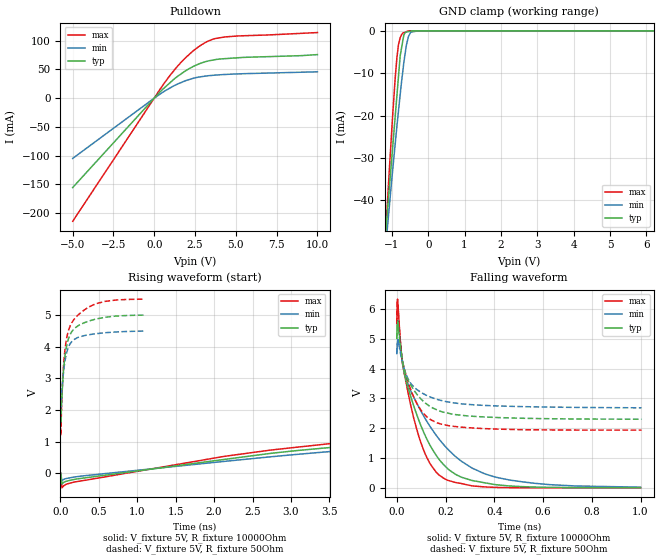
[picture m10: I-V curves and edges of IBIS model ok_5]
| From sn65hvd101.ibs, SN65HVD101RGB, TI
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|   ok_5 Model
[Model]   ok_5
Model_type   Open_drain
Polarity   Inverting
Vmeas = 2.5
Vref = 5
Cref = 2pF
Rref = 10000
|   typ   min   max
|   (nom PVT)   (fast PVT)   (slow PVT)
C_comp   1.593e-12   1.577e-12   1.617e-12
| Where nom  PVT is Nominal Process, 5V, 45C
|   Fast PVT is Strong Process,  5.5V, -20C
|   Slow PVT is Weak Process,   4.5V, 125C
[Voltage Range]   5   4.5   5.5
|Junction Temperature
[Temperature Range]   45   125   -20
[Pullup Reference]   5   4.5   5.5
[Pulldown Reference]   0   0   0
[Power Clamp Reference]   5   4.5   5.5
[GND Clamp Reference]   0   0   0
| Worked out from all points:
|   slope of the pulldown table from 0 to 0.75 V, typ, clamps not added: 35.3 ohm
|   GND clamp passes 1 mA (typ) near -0.67 V on its own axis
|   falling waveform, V_fixture 5V, R_fixture 10000Ohm: 20-80 % time 142ps typ, 220ps min, 98.9ps max; typ from 5 V to 0.017 V
|   rising waveform, V_fixture 5V, R_fixture 10000Ohm: 20-80 % time 27.8ns typ, 28.8ns min, 27.6ns max; typ from 0.016 V to 5 V
|   falling waveform, V_fixture 5V, R_fixture 50Ohm: 20-80 % time 97.8ps typ, 111ps min, 79.6ps max; typ from 5 V to 2.31 V
|   rising waveform, V_fixture 5V, R_fixture 50Ohm: 20-80 % time 115ps typ, 104ps min, 133ps max; typ from 2.31 V to 4.99 V
[Pulldown]
|   Voltage   I(typ)   I(min)   I(max)
-5V       -155.5mA   -104.9mA   -214.2mA
555.5mV   16.29mA    10.79mA    23.77mA
1.413V    37.57mA    24.3mA     55.1mA
1.875V    46.72mA    29.8mA     69.12mA
2.376V    54.89mA    34.39mA    82mA
2.811V    60.31mA    36.99mA    91.18mA
3.278V    64.46mA    38.86mA    98.87mA
3.735V    66.94mA    40.02mA    103.6mA
4.34V     68.66mA    41.14mA    106.5mA
10V       75.7mA     45.78mA    114mA
[GND Clamp]
|   Voltage   I(typ)   I(min)   I(max)
-5V       -440.9mA   -407.3mA   -496.8mA
-1.373V   -72.14mA   -70.31mA   -78.8mA
-1.14V    -44.59mA   -48.27mA   -43.57mA
-1.083V   -38.68mA   -42.92mA   -35.01mA
-984.5mV  -28.33mA   -33.6mA    -21.01mA
-913mV    -20.85mA   -27.23mA   -11.88mA
-858mV    -15.1mA    -22.33mA   -6.169mA
-770mV    -5.896mA   -15.04mA   -1.624mA
-670mV    -988.3uA   -7.517mA   -448.3uA
-544.5mV  -191.4uA   -1.37mA    -21.14uA
-274.5mV  -875.9nA   -1.632uA   -1.497uA
10V       0A         0A         0A
[POWER Clamp]
|   Voltage   I(typ)   I(min)   I(max)
-5V       0A         0A         0A
0V        0A         0A         0A
10V       0A         0A         0A
[Ramp]
R_load = 10000
|   typ   min   max
dV/dt_r   2.98901/2.77404e-08   2.68553/2.87811e-08   3.29113/2.74155e-08
dV/dt_f   2.98971/1.41722e-10   2.67881/2.19603e-10   3.2927/9.87492e-11
[Falling Waveform]
V_fixture = 5V
V_fixture_min = 4.5V
V_fixture_max = 5.5V
R_fixture = 10000Ohm
|   Time   V(typ)   V(min)   V(max)
0s        5V         4.5V       5.5V
3ps       5.598V     4.908V     6.318V
23ps      4.255V     4.251V     4.184V
48ps      3.318V     3.438V     3.126V
87ps      2.344V     2.762V     1.825V
134ps     1.471V     2.096V     858.5mV
190ps     805.2mV    1.478V     347.1mV
306ps     264.4mV    687.4mV    82.88mV
411ps     113.9mV    359.5mV    26.78mV
1ns       17.06mV    35.23mV    12.05mV
[Rising Waveform]
V_fixture = 5V
V_fixture_min = 4.5V
V_fixture_max = 5.5V
R_fixture = 10000Ohm
|   Time   V(typ)   V(min)   V(max)
0s        15.91mV    21.46mV    12.17mV
20ps      -341.8mV   -237.5mV   -461.1mV
2.12ns    432.4mV    371.4mV    528.2mV
3.84ns    873mV      747.2mV    1.01V
10.12ns   1.95V      1.681V     2.204V
16.76ns   2.807V     2.445V     3.142V
27.36ns   3.716V     3.274V     4.124V
40.14ns   4.33V      3.849V     4.783V
74.06ns   4.882V     4.38V      5.373V
150ns     4.998V     4.497V     5.497V
[Falling Waveform]
V_fixture = 5V
V_fixture_min = 4.5V
V_fixture_max = 5.5V
R_fixture = 50Ohm
|   Time   V(typ)   V(min)   V(max)
0s        5V         4.5V       5.5V
2ps       5.467V     4.792V     6.215V
4ps       5.567V     4.931V     6.189V
14ps      4.812V     4.554V     4.957V
24ps      4.24V      4.181V     4.227V
64ps      3.358V     3.437V     3.153V
106ps     2.926V     3.171V     2.535V
162ps     2.627V     2.976V     2.197V
372ps     2.376V     2.762V     1.988V
1.004ns   2.306V     2.687V     1.942V
[Rising Waveform]
V_fixture = 5V
V_fixture_min = 4.5V
V_fixture_max = 5.5V
R_fixture = 50Ohm
|   Time   V(typ)   V(min)   V(max)
0s        2.306V     2.68V      1.946V
2ps       1.827V     2.338V     1.354V
4ps       1.573V     2.119V     1.19V
18ps      2.354V     2.549V     2.33V
32ps      2.975V     2.996V     3.085V
70ps      3.884V     3.688V     4.108V
108ps     4.273V     4.003V     4.534V
172ps     4.544V     4.212V     4.844V
476ps     4.876V     4.41V      5.361V
1.096ns   4.994V     4.489V     5.497V
